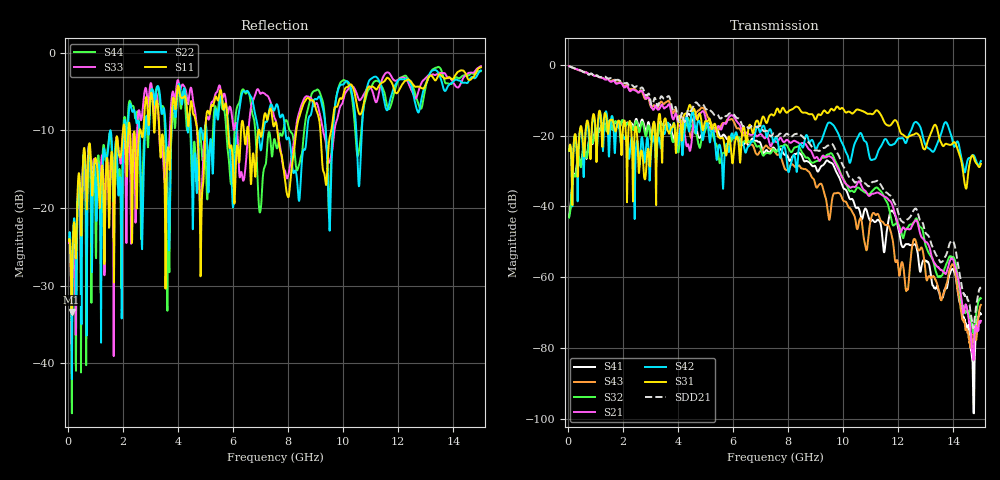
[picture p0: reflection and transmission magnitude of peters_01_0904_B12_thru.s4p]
# MHZ S RI R 50.00
! FREQ  S11  S12  S13  S14
!  S21  S22  S23  S24
!  S31  S32  S33  S34
!  S41  S42  S43  S44
!  REAL  IMAG  REAL  IMAG  REAL  IMAG  REAL  IMAG
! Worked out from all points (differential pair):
!   1496 points, 50 MHz to 15 GHz, reference 50 ohm
!   strongest paths, dB at 50 MHz, 3.79 GHz, 7.53 GHz, 11.27 GHz, 15 GHz:
!     S31: -24.3, -17.7, -13.7, -13.1, -28.0
!     S42: -24.3, -18.1, -20.7, -24.4, -27.2
!     S21: -0.4, -14.8, -21.5, -36.1, -72.3
!     S32: -43.1, -21.3, -24.5, -34.9, -65.9
!     S43: -0.4, -13.5, -24.7, -42.2, -67.8
!     S41: -42.9, -19.7, -23.9, -43.8, -70.4
!   taken as a pair (ports 1,3 in; 2,4 out), SDD21 dB: -0.4, -12.2, -19.8, -32.9, -62.8
!   lowest |S11| = -33.4 dB at 140 MHz (marker M1), VSWR 1.04, Z = 52.2 - j0.0314 ohm
!   |S11| at or under -10 dB: start of sweep to 2.008 GHz; 5.824 GHz to 6.292 GHz (468.7 MHz wide, 7.74 % of centre); 7.61 GHz to 8.302 GHz (692.9 MHz wide, 8.71 % of centre)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
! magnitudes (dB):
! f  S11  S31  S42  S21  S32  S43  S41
! 50 MHz  -24.3  -24.3  -24.3  -0.4  -43.1  -0.4  -42.9
! 140 MHz  -33.4  -28.7  -28.9  -0.7  -35.9  -0.7  -35.7
! 1.28 GHz  -16.0  -19.8  -24.4  -3.8  -16.5  -3.8  -16.5
! 2.8 GHz  -7.0  -32.4  -27.1  -9.1  -19.3  -9.6  -17.9
! 4.41 GHz  -8.5  -11.5  -18.9  -23.7  -15.9  -18.5  -13.9
! 9.55 GHz  -10.3  -12.5  -16.4  -26.0  -25.0  -41.0  -27.6
! 15 GHz  -1.9  -28.0  -27.2  -72.3  -65.9  -67.8  -70.4
